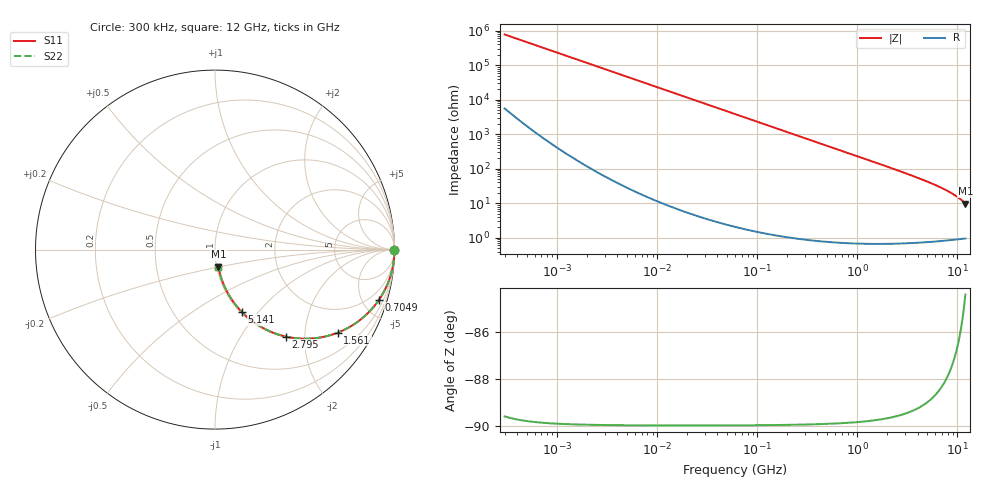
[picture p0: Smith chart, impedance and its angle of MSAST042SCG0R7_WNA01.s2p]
! MSAST042SCG0R7_WNA01  S-PARAMETER MODEL  ( General Type )
! Model Generated by TAIYO YUDEN Corporation (http://www.ty-top.com)
! Version 1.0
! TAIYO YUDEN Control No. 150820
! Copyright(c) 2015 TAIYO YUDEN CO.,LTD. All Rights Reserved.
! Product Description (link to TY-COMPAS)
! https://ds.yuden.co.jp/TYCOMPAS/or/detail?pn=MSAST042SCG0R7AWNA01&u=M
! Products Name : Multilayer Ceramic Capacitors
! Characteristics :
!  Capacitance : 0.7 pF , Rated Voltage : 25V , TCC : CG / C0G
!  Case Size : 0.4 x 0.2 / 0.016 x 0.008 [mm/inch] , Thickness : 0.2 / 0.008 [mm/inch]
!  (Conditions: Temperature = 25 degC , DC Bias Current/Voltage = 0A / 0V)
! External Node Assignments :
!  1  o---| |---o  2
! GND o---------o GND
! Frequency Range : 0.3MHz  -  12000MHz  [ 401 STEP ]
# MHz S RI R 50
! Freq[MHz].  S11 Real  S11 Imag  S21 Real  S21 Imag  S12 Real  S12 Imag  S22 Real  S22 Imag
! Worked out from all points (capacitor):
!   401 points, 300 kHz to 12 GHz, reference 50 ohm
!   read as one part in series: C = 686 fF near 316.3 kHz
!   lowest |Z| = 9.81 ohm at 12 GHz (marker M1)
!   S11 on the Smith chart (normalised r, x): 300 kHz: open; 704.9 MHz: 1.01, -6.58; 1.561 GHz: 1.01, -2.95; 2.795 GHz: 1.01, -1.62; 5.141 GHz: 1.02, -0.82; 12 GHz: 1.02, -0.20
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0.3  1 -0.000129  9.48e-07 0.000129  9.48e-07 0.000129  1 -0.000129
0.316324  1 -0.000136  9.31e-07 0.000136  9.31e-07 0.000136  1 -0.000136
1.769972  1 -0.000762  1.42e-06 0.000762  1.42e-06 0.000762  1 -0.000762
10.44266  1 -0.0045  2.24e-05 0.0045  2.24e-05 0.0045  1 -0.0045
60  0.9993 -0.0258  0.000681 0.0258  0.000681 0.0258  0.9993 -0.0258
164.1901  0.995 -0.0704  0.00503 0.0704  0.00503 0.0704  0.995 -0.0704
244.3004  0.9889 -0.1041  0.0111 0.1041  0.0111 0.1041  0.9889 -0.1041
353.9943  0.9771 -0.149  0.0229 0.149  0.0229 0.149  0.9771 -0.149
512.9422  0.9531 -0.2107  0.0469 0.2107  0.0469 0.2107  0.9531 -0.2107
704.9044  0.9148 -0.2781  0.0852 0.2781  0.0852 0.2781  0.9148 -0.2781
1048.836  0.8287 -0.3753  0.1713 0.3753  0.1713 0.3753  0.8287 -0.3753
1262.535  0.769 -0.4197  0.231 0.4197  0.231 0.4197  0.769 -0.4197
1560.575  0.6844 -0.4625  0.3156 0.4625  0.3156 0.4625  0.6844 -0.4625
2088.533  0.5449 -0.4949  0.4551 0.4949  0.4551 0.4949  0.5449 -0.4949
2795.104  0.396 -0.4848  0.604 0.4848  0.604 0.4848  0.396 -0.4848
3841.137  0.2503 -0.427  0.7497 0.427  0.7497 0.427  0.2503 -0.427
5140.631  0.1488 -0.3468  0.8512 0.3468  0.8512 0.3468  0.1488 -0.3468
6699.894  0.0852 -0.2659  0.9148 0.2659  0.9148 0.2659  0.0852 -0.2659
8281.503  0.0512 -0.2015  0.9488 0.2015  0.9488 0.2015  0.0512 -0.2015
9708.23  0.0336 -0.1548  0.9664 0.1548  0.9664 0.1548  0.0336 -0.1548
11380.75  0.0216 -0.1096  0.9784 0.1096  0.9784 0.1096  0.0216 -0.1096
12000  0.0186 -0.0949  0.9814 0.0949  0.9814 0.0949  0.0186 -0.0949
